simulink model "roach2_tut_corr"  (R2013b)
settings: Solver=VariableStepDiscrete  SolverMode=SingleTasking  StartTime=0.0  StopTime=100  RelTol=1e-3
undefined symbols (not defined in the file): add_latency, addr_width, Bit, bitfield, BitWidth, bram_latency, burst_size, casper_library_scopes, conv_latency, data_width, DelayLen, fan_latency, FFTSize, FFTStage, getfield, increment, led, Location, Lower, mult_latency, mux_latency, n_bits, n_bits_data, n_inputs, n_streams, n_taps, neg_latency, negate_latency, nsamples, pfb_size, pulse_len, reset_period, ROACH, ROACH2, snapshot, sx475t, sync_period, sync_period_bits, Upper, UseCounter, Width
libraries: xbsIndex_r4 x24444, casper_library_misc x73, xbsReplacements_r4 x34, casper_library_delays x14, xps_library x7
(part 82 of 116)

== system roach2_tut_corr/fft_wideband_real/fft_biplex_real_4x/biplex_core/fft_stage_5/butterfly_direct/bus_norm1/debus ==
  bus_in : Inport
  reinterpret{1..16} (16 alike) : xbsIndex_r4/Reinterpret  force_arith_type=on  arith_type="Signed  (2's comp)"  force_bin_pt=on  bin_pt=18  block_type=reinterpret
  slice1 : xbsIndex_r4/Slice  nbits=20  boolean_output=off  mode=Upper Bit Location + Width  bit1=-300  base1=MSB of Input  bit0=0  base0=LSB of Input  dbl_ovrd=off  block_type=slice
  slice10 : xbsIndex_r4/Slice  nbits=20  boolean_output=off  mode=Upper Bit Location + Width  bit1=-120  base1=MSB of Input  bit0=0  base0=LSB of Input  dbl_ovrd=off  block_type=slice
  slice11 : xbsIndex_r4/Slice  nbits=20  boolean_output=off  mode=Upper Bit Location + Width  bit1=-100  base1=MSB of Input  bit0=0  base0=LSB of Input  dbl_ovrd=off  block_type=slice
  slice12 : xbsIndex_r4/Slice  nbits=20  boolean_output=off  mode=Upper Bit Location + Width  bit1=-80  base1=MSB of Input  bit0=0  base0=LSB of Input  dbl_ovrd=off  block_type=slice
  slice13 : xbsIndex_r4/Slice  nbits=20  boolean_output=off  mode=Upper Bit Location + Width  bit1=-60  base1=MSB of Input  bit0=0  base0=LSB of Input  dbl_ovrd=off  block_type=slice
  slice14 : xbsIndex_r4/Slice  nbits=20  boolean_output=off  mode=Upper Bit Location + Width  bit1=-40  base1=MSB of Input  bit0=0  base0=LSB of Input  dbl_ovrd=off  block_type=slice
  slice15 : xbsIndex_r4/Slice  nbits=20  boolean_output=off  mode=Upper Bit Location + Width  bit1=-20  base1=MSB of Input  bit0=0  base0=LSB of Input  dbl_ovrd=off  block_type=slice
  slice16 : xbsIndex_r4/Slice  nbits=20  boolean_output=off  mode=Upper Bit Location + Width  bit1=0  base1=MSB of Input  bit0=0  base0=LSB of Input  dbl_ovrd=off  block_type=slice
  slice2 : xbsIndex_r4/Slice  nbits=20  boolean_output=off  mode=Upper Bit Location + Width  bit1=-280  base1=MSB of Input  bit0=0  base0=LSB of Input  dbl_ovrd=off  block_type=slice
  slice3 : xbsIndex_r4/Slice  nbits=20  boolean_output=off  mode=Upper Bit Location + Width  bit1=-260  base1=MSB of Input  bit0=0  base0=LSB of Input  dbl_ovrd=off  block_type=slice
  slice4 : xbsIndex_r4/Slice  nbits=20  boolean_output=off  mode=Upper Bit Location + Width  bit1=-240  base1=MSB of Input  bit0=0  base0=LSB of Input  dbl_ovrd=off  block_type=slice
  slice5 : xbsIndex_r4/Slice  nbits=20  boolean_output=off  mode=Upper Bit Location + Width  bit1=-220  base1=MSB of Input  bit0=0  base0=LSB of Input  dbl_ovrd=off  block_type=slice
  slice6 : xbsIndex_r4/Slice  nbits=20  boolean_output=off  mode=Upper Bit Location + Width  bit1=-200  base1=MSB of Input  bit0=0  base0=LSB of Input  dbl_ovrd=off  block_type=slice
  slice7 : xbsIndex_r4/Slice  nbits=20  boolean_output=off  mode=Upper Bit Location + Width  bit1=-180  base1=MSB of Input  bit0=0  base0=LSB of Input  dbl_ovrd=off  block_type=slice
  slice8 : xbsIndex_r4/Slice  nbits=20  boolean_output=off  mode=Upper Bit Location + Width  bit1=-160  base1=MSB of Input  bit0=0  base0=LSB of Input  dbl_ovrd=off  block_type=slice
  slice9 : xbsIndex_r4/Slice  nbits=20  boolean_output=off  mode=Upper Bit Location + Width  bit1=-140  base1=MSB of Input  bit0=0  base0=LSB of Input  dbl_ovrd=off  block_type=slice
  msb_out16 : Outport
  out15 : Outport  Port=2
  out14 : Outport  Port=3
  out13 : Outport  Port=4
  out12 : Outport  Port=5
  out11 : Outport  Port=6
  out10 : Outport  Port=7
  out9 : Outport  Port=8
  out8 : Outport  Port=9
  out7 : Outport  Port=10
  out6 : Outport  Port=11
  out5 : Outport  Port=12
  out4 : Outport  Port=13
  out3 : Outport  Port=14
  out2 : Outport  Port=15
  lsb_out1 : Outport  Port=16
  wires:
  bus_in/1 -> slice16/1, slice15/1, slice14/1, slice13/1, slice12/1, slice11/1, slice10/1, slice9/1, slice8/1, slice7/1, slice6/1, slice5/1, slice4/1, slice3/1, slice2/1, slice1/1
  slice16/1 -> reinterpret16/1
  reinterpret16/1 -> msb_out16/1
  slice15/1 -> reinterpret15/1
  reinterpret15/1 -> out15/1
  slice14/1 -> reinterpret14/1
  reinterpret14/1 -> out14/1
  slice13/1 -> reinterpret13/1
  reinterpret13/1 -> out13/1
  slice12/1 -> reinterpret12/1
  reinterpret12/1 -> out12/1
  slice11/1 -> reinterpret11/1
  reinterpret11/1 -> out11/1
  slice10/1 -> reinterpret10/1
  reinterpret10/1 -> out10/1
  slice9/1 -> reinterpret9/1
  reinterpret9/1 -> out9/1
  slice8/1 -> reinterpret8/1
  reinterpret8/1 -> out8/1
  slice7/1 -> reinterpret7/1
  reinterpret7/1 -> out7/1
  slice6/1 -> reinterpret6/1
  reinterpret6/1 -> out6/1
  slice5/1 -> reinterpret5/1
  reinterpret5/1 -> out5/1
  slice4/1 -> reinterpret4/1
  reinterpret4/1 -> out4/1
  slice3/1 -> reinterpret3/1
  reinterpret3/1 -> out3/1
  slice2/1 -> reinterpret2/1
  reinterpret2/1 -> out2/1
  slice1/1 -> reinterpret1/1
  reinterpret1/1 -> lsb_out1/1

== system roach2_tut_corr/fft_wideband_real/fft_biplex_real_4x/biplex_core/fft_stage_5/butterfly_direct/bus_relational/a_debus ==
  bus_in : Inport
  reinterpret1 : xbsIndex_r4/Reinterpret  force_arith_type=on  arith_type=Unsigned  force_bin_pt=on  bin_pt=0  block_type=reinterpret
  slice1 : xbsIndex_r4/Slice  nbits=4  boolean_output=off  mode=Upper Bit Location + Width  bit1=0  base1=MSB of Input  bit0=0  base0=LSB of Input  dbl_ovrd=off  block_type=slice
  msb_lsb_out1 : Outport
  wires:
  bus_in/1 -> slice1/1
  slice1/1 -> reinterpret1/1
  reinterpret1/1 -> msb_lsb_out1/1

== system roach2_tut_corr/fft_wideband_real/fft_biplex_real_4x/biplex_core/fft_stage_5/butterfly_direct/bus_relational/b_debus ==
  bus_in : Inport
  reinterpret{1..4} (4 alike) : xbsIndex_r4/Reinterpret  force_arith_type=on  arith_type=Unsigned  force_bin_pt=on  bin_pt=0  block_type=reinterpret
  slice1 : xbsIndex_r4/Slice  nbits=4  boolean_output=off  mode=Upper Bit Location + Width  bit1=-12  base1=MSB of Input  bit0=0  base0=LSB of Input  dbl_ovrd=off  block_type=slice
  slice2 : xbsIndex_r4/Slice  nbits=4  boolean_output=off  mode=Upper Bit Location + Width  bit1=-8  base1=MSB of Input  bit0=0  base0=LSB of Input  dbl_ovrd=off  block_type=slice
  slice3 : xbsIndex_r4/Slice  nbits=4  boolean_output=off  mode=Upper Bit Location + Width  bit1=-4  base1=MSB of Input  bit0=0  base0=LSB of Input  dbl_ovrd=off  block_type=slice
  slice4 : xbsIndex_r4/Slice  nbits=4  boolean_output=off  mode=Upper Bit Location + Width  bit1=0  base1=MSB of Input  bit0=0  base0=LSB of Input  dbl_ovrd=off  block_type=slice
  msb_out4 : Outport
  out3 : Outport  Port=2
  out2 : Outport  Port=3
  lsb_out1 : Outport  Port=4
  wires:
  bus_in/1 -> slice4/1, slice3/1, slice2/1, slice1/1
  slice4/1 -> reinterpret4/1
  reinterpret4/1 -> msb_out4/1
  slice3/1 -> reinterpret3/1
  reinterpret3/1 -> out3/1
  slice2/1 -> reinterpret2/1
  reinterpret2/1 -> out2/1
  slice1/1 -> reinterpret1/1
  reinterpret1/1 -> lsb_out1/1

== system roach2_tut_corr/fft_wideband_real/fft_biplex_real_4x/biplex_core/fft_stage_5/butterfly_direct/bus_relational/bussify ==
  in1 : Inport
  in2 : Inport  Port=2
  in3 : Inport  Port=3
  in4 : Inport  Port=4
  concatenate : xbsIndex_r4/Concat  num_inputs=4  dbl_ovrd=off  block_type=concat
  reinterpret{1..4} (4 alike) : xbsIndex_r4/Reinterpret  force_arith_type=on  arith_type=Unsigned  force_bin_pt=on  bin_pt=0  block_type=reinterpret
  bus_out : Outport
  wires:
  concatenate/1 -> bus_out/1
  in1/1 -> reinterpret1/1
  reinterpret1/1 -> concatenate/1
  in2/1 -> reinterpret2/1
  reinterpret2/1 -> concatenate/2
  in3/1 -> reinterpret3/1
  reinterpret3/1 -> concatenate/3
  in4/1 -> reinterpret4/1
  reinterpret4/1 -> concatenate/4

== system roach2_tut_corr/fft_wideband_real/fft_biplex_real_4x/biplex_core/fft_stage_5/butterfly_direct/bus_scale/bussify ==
  in1 : Inport
  in2 : Inport  Port=2
  in3 : Inport  Port=3
  in4 : Inport  Port=4
  in5 : Inport  Port=5
  in6 : Inport  Port=6
  in7 : Inport  Port=7
  in8 : Inport  Port=8
  in9 : Inport  Port=9
  in10 : Inport  Port=10
  in11 : Inport  Port=11
  in12 : Inport  Port=12
  in13 : Inport  Port=13
  in14 : Inport  Port=14
  in15 : Inport  Port=15
  in16 : Inport  Port=16
  concatenate : xbsIndex_r4/Concat  num_inputs=16  dbl_ovrd=off  block_type=concat
  reinterpret{1..16} (16 alike) : xbsIndex_r4/Reinterpret  force_arith_type=on  arith_type=Unsigned  force_bin_pt=on  bin_pt=0  block_type=reinterpret
  bus_out : Outport
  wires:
  concatenate/1 -> bus_out/1
  in1/1 -> reinterpret1/1
  reinterpret1/1 -> concatenate/1
  in2/1 -> reinterpret2/1
  reinterpret2/1 -> concatenate/2
  in3/1 -> reinterpret3/1
  reinterpret3/1 -> concatenate/3
  in4/1 -> reinterpret4/1
  reinterpret4/1 -> concatenate/4
  in5/1 -> reinterpret5/1
  reinterpret5/1 -> concatenate/5
  in6/1 -> reinterpret6/1
  reinterpret6/1 -> concatenate/6
  in7/1 -> reinterpret7/1
  reinterpret7/1 -> concatenate/7
  in8/1 -> reinterpret8/1
  reinterpret8/1 -> concatenate/8
  in9/1 -> reinterpret9/1
  reinterpret9/1 -> concatenate/9
  in10/1 -> reinterpret10/1
  reinterpret10/1 -> concatenate/10
  in11/1 -> reinterpret11/1
  reinterpret11/1 -> concatenate/11
  in12/1 -> reinterpret12/1
  reinterpret12/1 -> concatenate/12
  in13/1 -> reinterpret13/1
  reinterpret13/1 -> concatenate/13
  in14/1 -> reinterpret14/1
  reinterpret14/1 -> concatenate/14
  in15/1 -> reinterpret15/1
  reinterpret15/1 -> concatenate/15
  in16/1 -> reinterpret16/1
  reinterpret16/1 -> concatenate/16

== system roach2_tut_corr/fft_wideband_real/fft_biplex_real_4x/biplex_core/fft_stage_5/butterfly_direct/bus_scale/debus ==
  bus_in : Inport
  reinterpret{1..16} (16 alike) : xbsIndex_r4/Reinterpret  force_arith_type=on  arith_type="Signed  (2's comp)"  force_bin_pt=on  bin_pt=17  block_type=reinterpret
  slice1 : xbsIndex_r4/Slice  nbits=20  boolean_output=off  mode=Upper Bit Location + Width  bit1=-300  base1=MSB of Input  bit0=0  base0=LSB of Input  dbl_ovrd=off  block_type=slice
  slice10 : xbsIndex_r4/Slice  nbits=20  boolean_output=off  mode=Upper Bit Location + Width  bit1=-120  base1=MSB of Input  bit0=0  base0=LSB of Input  dbl_ovrd=off  block_type=slice
  slice11 : xbsIndex_r4/Slice  nbits=20  boolean_output=off  mode=Upper Bit Location + Width  bit1=-100  base1=MSB of Input  bit0=0  base0=LSB of Input  dbl_ovrd=off  block_type=slice
  slice12 : xbsIndex_r4/Slice  nbits=20  boolean_output=off  mode=Upper Bit Location + Width  bit1=-80  base1=MSB of Input  bit0=0  base0=LSB of Input  dbl_ovrd=off  block_type=slice
  slice13 : xbsIndex_r4/Slice  nbits=20  boolean_output=off  mode=Upper Bit Location + Width  bit1=-60  base1=MSB of Input  bit0=0  base0=LSB of Input  dbl_ovrd=off  block_type=slice
  slice14 : xbsIndex_r4/Slice  nbits=20  boolean_output=off  mode=Upper Bit Location + Width  bit1=-40  base1=MSB of Input  bit0=0  base0=LSB of Input  dbl_ovrd=off  block_type=slice
  slice15 : xbsIndex_r4/Slice  nbits=20  boolean_output=off  mode=Upper Bit Location + Width  bit1=-20  base1=MSB of Input  bit0=0  base0=LSB of Input  dbl_ovrd=off  block_type=slice
  slice16 : xbsIndex_r4/Slice  nbits=20  boolean_output=off  mode=Upper Bit Location + Width  bit1=0  base1=MSB of Input  bit0=0  base0=LSB of Input  dbl_ovrd=off  block_type=slice
  slice2 : xbsIndex_r4/Slice  nbits=20  boolean_output=off  mode=Upper Bit Location + Width  bit1=-280  base1=MSB of Input  bit0=0  base0=LSB of Input  dbl_ovrd=off  block_type=slice
  slice3 : xbsIndex_r4/Slice  nbits=20  boolean_output=off  mode=Upper Bit Location + Width  bit1=-260  base1=MSB of Input  bit0=0  base0=LSB of Input  dbl_ovrd=off  block_type=slice
  slice4 : xbsIndex_r4/Slice  nbits=20  boolean_output=off  mode=Upper Bit Location + Width  bit1=-240  base1=MSB of Input  bit0=0  base0=LSB of Input  dbl_ovrd=off  block_type=slice
  slice5 : xbsIndex_r4/Slice  nbits=20  boolean_output=off  mode=Upper Bit Location + Width  bit1=-220  base1=MSB of Input  bit0=0  base0=LSB of Input  dbl_ovrd=off  block_type=slice
  slice6 : xbsIndex_r4/Slice  nbits=20  boolean_output=off  mode=Upper Bit Location + Width  bit1=-200  base1=MSB of Input  bit0=0  base0=LSB of Input  dbl_ovrd=off  block_type=slice
  slice7 : xbsIndex_r4/Slice  nbits=20  boolean_output=off  mode=Upper Bit Location + Width  bit1=-180  base1=MSB of Input  bit0=0  base0=LSB of Input  dbl_ovrd=off  block_type=slice
  slice8 : xbsIndex_r4/Slice  nbits=20  boolean_output=off  mode=Upper Bit Location + Width  bit1=-160  base1=MSB of Input  bit0=0  base0=LSB of Input  dbl_ovrd=off  block_type=slice
  slice9 : xbsIndex_r4/Slice  nbits=20  boolean_output=off  mode=Upper Bit Location + Width  bit1=-140  base1=MSB of Input  bit0=0  base0=LSB of Input  dbl_ovrd=off  block_type=slice
  msb_out16 : Outport
  out15 : Outport  Port=2
  out14 : Outport  Port=3
  out13 : Outport  Port=4
  out12 : Outport  Port=5
  out11 : Outport  Port=6
  out10 : Outport  Port=7
  out9 : Outport  Port=8
  out8 : Outport  Port=9
  out7 : Outport  Port=10
  out6 : Outport  Port=11
  out5 : Outport  Port=12
  out4 : Outport  Port=13
  out3 : Outport  Port=14
  out2 : Outport  Port=15
  lsb_out1 : Outport  Port=16
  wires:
  bus_in/1 -> slice16/1, slice15/1, slice14/1, slice13/1, slice12/1, slice11/1, slice10/1, slice9/1, slice8/1, slice7/1, slice6/1, slice5/1, slice4/1, slice3/1, slice2/1, slice1/1
  slice16/1 -> reinterpret16/1
  reinterpret16/1 -> msb_out16/1
  slice15/1 -> reinterpret15/1
  reinterpret15/1 -> out15/1
  slice14/1 -> reinterpret14/1
  reinterpret14/1 -> out14/1
  slice13/1 -> reinterpret13/1
  reinterpret13/1 -> out13/1
  slice12/1 -> reinterpret12/1
  reinterpret12/1 -> out12/1
  slice11/1 -> reinterpret11/1
  reinterpret11/1 -> out11/1
  slice10/1 -> reinterpret10/1
  reinterpret10/1 -> out10/1
  slice9/1 -> reinterpret9/1
  reinterpret9/1 -> out9/1
  slice8/1 -> reinterpret8/1
  reinterpret8/1 -> out8/1
  slice7/1 -> reinterpret7/1
  reinterpret7/1 -> out7/1
  slice6/1 -> reinterpret6/1
  reinterpret6/1 -> out6/1
  slice5/1 -> reinterpret5/1
  reinterpret5/1 -> out5/1
  slice4/1 -> reinterpret4/1
  reinterpret4/1 -> out4/1
  slice3/1 -> reinterpret3/1
  reinterpret3/1 -> out3/1
  slice2/1 -> reinterpret2/1
  reinterpret2/1 -> out2/1
  slice1/1 -> reinterpret1/1
  reinterpret1/1 -> lsb_out1/1

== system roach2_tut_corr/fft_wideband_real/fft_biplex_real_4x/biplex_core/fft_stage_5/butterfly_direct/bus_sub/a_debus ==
  bus_in : Inport
  reinterpret{1..8} (8 alike) : xbsIndex_r4/Reinterpret  force_arith_type=on  arith_type="Signed  (2's comp)"  force_bin_pt=on  bin_pt=17  block_type=reinterpret
  slice1 : xbsIndex_r4/Slice  nbits=18  boolean_output=off  mode=Upper Bit Location + Width  bit1=-126  base1=MSB of Input  bit0=0  base0=LSB of Input  dbl_ovrd=off  block_type=slice
  slice2 : xbsIndex_r4/Slice  nbits=18  boolean_output=off  mode=Upper Bit Location + Width  bit1=-108  base1=MSB of Input  bit0=0  base0=LSB of Input  dbl_ovrd=off  block_type=slice
  slice3 : xbsIndex_r4/Slice  nbits=18  boolean_output=off  mode=Upper Bit Location + Width  bit1=-90  base1=MSB of Input  bit0=0  base0=LSB of Input  dbl_ovrd=off  block_type=slice
  slice4 : xbsIndex_r4/Slice  nbits=18  boolean_output=off  mode=Upper Bit Location + Width  bit1=-72  base1=MSB of Input  bit0=0  base0=LSB of Input  dbl_ovrd=off  block_type=slice
  slice5 : xbsIndex_r4/Slice  nbits=18  boolean_output=off  mode=Upper Bit Location + Width  bit1=-54  base1=MSB of Input  bit0=0  base0=LSB of Input  dbl_ovrd=off  block_type=slice
  slice6 : xbsIndex_r4/Slice  nbits=18  boolean_output=off  mode=Upper Bit Location + Width  bit1=-36  base1=MSB of Input  bit0=0  base0=LSB of Input  dbl_ovrd=off  block_type=slice
  slice7 : xbsIndex_r4/Slice  nbits=18  boolean_output=off  mode=Upper Bit Location + Width  bit1=-18  base1=MSB of Input  bit0=0  base0=LSB of Input  dbl_ovrd=off  block_type=slice
  slice8 : xbsIndex_r4/Slice  nbits=18  boolean_output=off  mode=Upper Bit Location + Width  bit1=0  base1=MSB of Input  bit0=0  base0=LSB of Input  dbl_ovrd=off  block_type=slice
  msb_out8 : Outport
  out7 : Outport  Port=2
  out6 : Outport  Port=3
  out5 : Outport  Port=4
  out4 : Outport  Port=5
  out3 : Outport  Port=6
  out2 : Outport  Port=7
  lsb_out1 : Outport  Port=8
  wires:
  bus_in/1 -> slice8/1, slice7/1, slice6/1, slice5/1, slice4/1, slice3/1, slice2/1, slice1/1
  slice8/1 -> reinterpret8/1
  reinterpret8/1 -> msb_out8/1
  slice7/1 -> reinterpret7/1
  reinterpret7/1 -> out7/1
  slice6/1 -> reinterpret6/1
  reinterpret6/1 -> out6/1
  slice5/1 -> reinterpret5/1
  reinterpret5/1 -> out5/1
  slice4/1 -> reinterpret4/1
  reinterpret4/1 -> out4/1
  slice3/1 -> reinterpret3/1
  reinterpret3/1 -> out3/1
  slice2/1 -> reinterpret2/1
  reinterpret2/1 -> out2/1
  slice1/1 -> reinterpret1/1
  reinterpret1/1 -> lsb_out1/1

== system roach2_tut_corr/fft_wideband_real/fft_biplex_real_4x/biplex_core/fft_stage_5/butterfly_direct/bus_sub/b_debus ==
  bus_in : Inport
  reinterpret{1..8} (8 alike) : xbsIndex_r4/Reinterpret  force_arith_type=on  arith_type="Signed  (2's comp)"  force_bin_pt=on  bin_pt=17  block_type=reinterpret
  slice1 : xbsIndex_r4/Slice  nbits=19  boolean_output=off  mode=Upper Bit Location + Width  bit1=-133  base1=MSB of Input  bit0=0  base0=LSB of Input  dbl_ovrd=off  block_type=slice
  slice2 : xbsIndex_r4/Slice  nbits=19  boolean_output=off  mode=Upper Bit Location + Width  bit1=-114  base1=MSB of Input  bit0=0  base0=LSB of Input  dbl_ovrd=off  block_type=slice
  slice3 : xbsIndex_r4/Slice  nbits=19  boolean_output=off  mode=Upper Bit Location + Width  bit1=-95  base1=MSB of Input  bit0=0  base0=LSB of Input  dbl_ovrd=off  block_type=slice
  slice4 : xbsIndex_r4/Slice  nbits=19  boolean_output=off  mode=Upper Bit Location + Width  bit1=-76  base1=MSB of Input  bit0=0  base0=LSB of Input  dbl_ovrd=off  block_type=slice
  slice5 : xbsIndex_r4/Slice  nbits=19  boolean_output=off  mode=Upper Bit Location + Width  bit1=-57  base1=MSB of Input  bit0=0  base0=LSB of Input  dbl_ovrd=off  block_type=slice
  slice6 : xbsIndex_r4/Slice  nbits=19  boolean_output=off  mode=Upper Bit Location + Width  bit1=-38  base1=MSB of Input  bit0=0  base0=LSB of Input  dbl_ovrd=off  block_type=slice
  slice7 : xbsIndex_r4/Slice  nbits=19  boolean_output=off  mode=Upper Bit Location + Width  bit1=-19  base1=MSB of Input  bit0=0  base0=LSB of Input  dbl_ovrd=off  block_type=slice
  slice8 : xbsIndex_r4/Slice  nbits=19  boolean_output=off  mode=Upper Bit Location + Width  bit1=0  base1=MSB of Input  bit0=0  base0=LSB of Input  dbl_ovrd=off  block_type=slice
  msb_out8 : Outport
  out7 : Outport  Port=2
  out6 : Outport  Port=3
  out5 : Outport  Port=4
  out4 : Outport  Port=5
  out3 : Outport  Port=6
  out2 : Outport  Port=7
  lsb_out1 : Outport  Port=8
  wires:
  bus_in/1 -> slice8/1, slice7/1, slice6/1, slice5/1, slice4/1, slice3/1, slice2/1, slice1/1
  slice8/1 -> reinterpret8/1
  reinterpret8/1 -> msb_out8/1
  slice7/1 -> reinterpret7/1
  reinterpret7/1 -> out7/1
  slice6/1 -> reinterpret6/1
  reinterpret6/1 -> out6/1
  slice5/1 -> reinterpret5/1
  reinterpret5/1 -> out5/1
  slice4/1 -> reinterpret4/1
  reinterpret4/1 -> out4/1
  slice3/1 -> reinterpret3/1
  reinterpret3/1 -> out3/1
  slice2/1 -> reinterpret2/1
  reinterpret2/1 -> out2/1
  slice1/1 -> reinterpret1/1
  reinterpret1/1 -> lsb_out1/1

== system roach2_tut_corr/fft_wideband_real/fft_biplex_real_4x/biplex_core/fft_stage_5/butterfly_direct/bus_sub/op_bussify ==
  in1 : Inport
  in2 : Inport  Port=2
  in3 : Inport  Port=3
  in4 : Inport  Port=4
  in5 : Inport  Port=5
  in6 : Inport  Port=6
  in7 : Inport  Port=7
  in8 : Inport  Port=8
  concatenate : xbsIndex_r4/Concat  num_inputs=8  dbl_ovrd=off  block_type=concat
  reinterpret{1..8} (8 alike) : xbsIndex_r4/Reinterpret  force_arith_type=on  arith_type=Unsigned  force_bin_pt=on  bin_pt=0  block_type=reinterpret
  bus_out : Outport
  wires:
  concatenate/1 -> bus_out/1
  in1/1 -> reinterpret1/1
  reinterpret1/1 -> concatenate/1
  in2/1 -> reinterpret2/1
  reinterpret2/1 -> concatenate/2
  in3/1 -> reinterpret3/1
  reinterpret3/1 -> concatenate/3
  in4/1 -> reinterpret4/1
  reinterpret4/1 -> concatenate/4
  in5/1 -> reinterpret5/1
  reinterpret5/1 -> concatenate/5
  in6/1 -> reinterpret6/1
  reinterpret6/1 -> concatenate/6
  in7/1 -> reinterpret7/1
  reinterpret7/1 -> concatenate/7
  in8/1 -> reinterpret8/1
  reinterpret8/1 -> concatenate/8

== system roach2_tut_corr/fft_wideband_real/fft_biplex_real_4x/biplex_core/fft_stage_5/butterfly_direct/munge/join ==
  in1 : Inport
  in2 : Inport  Port=2
  in3 : Inport  Port=3
  in4 : Inport  Port=4
  in5 : Inport  Port=5
  in6 : Inport  Port=6
  in7 : Inport  Port=7
  in8 : Inport  Port=8
  concatenate : xbsIndex_r4/Concat  num_inputs=8  dbl_ovrd=off  block_type=concat
  reinterpret{1..8} (8 alike) : xbsIndex_r4/Reinterpret  force_arith_type=on  arith_type=Unsigned  force_bin_pt=on  bin_pt=0  block_type=reinterpret
  bus_out : Outport
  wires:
  concatenate/1 -> bus_out/1
  in1/1 -> reinterpret1/1
  reinterpret1/1 -> concatenate/1
  in2/1 -> reinterpret2/1
  reinterpret2/1 -> concatenate/2
  in3/1 -> reinterpret3/1
  reinterpret3/1 -> concatenate/3
  in4/1 -> reinterpret4/1
  reinterpret4/1 -> concatenate/4
  in5/1 -> reinterpret5/1
  reinterpret5/1 -> concatenate/5
  in6/1 -> reinterpret6/1
  reinterpret6/1 -> concatenate/6
  in7/1 -> reinterpret7/1
  reinterpret7/1 -> concatenate/7
  in8/1 -> reinterpret8/1
  reinterpret8/1 -> concatenate/8

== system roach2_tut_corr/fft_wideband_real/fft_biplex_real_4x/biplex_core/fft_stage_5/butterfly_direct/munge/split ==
  bus_in : Inport
  reinterpret{1..8} (8 alike) : xbsIndex_r4/Reinterpret  force_arith_type=on  arith_type=Unsigned  force_bin_pt=on  bin_pt=0  block_type=reinterpret
  slice1 : xbsIndex_r4/Slice  nbits=2  boolean_output=off  mode=Upper Bit Location + Width  bit1=-14  base1=MSB of Input  bit0=0  base0=LSB of Input  dbl_ovrd=off  block_type=slice
  slice2 : xbsIndex_r4/Slice  nbits=2  boolean_output=off  mode=Upper Bit Location + Width  bit1=-12  base1=MSB of Input  bit0=0  base0=LSB of Input  dbl_ovrd=off  block_type=slice
  slice3 : xbsIndex_r4/Slice  nbits=2  boolean_output=off  mode=Upper Bit Location + Width  bit1=-10  base1=MSB of Input  bit0=0  base0=LSB of Input  dbl_ovrd=off  block_type=slice
  slice4 : xbsIndex_r4/Slice  nbits=2  boolean_output=off  mode=Upper Bit Location + Width  bit1=-8  base1=MSB of Input  bit0=0  base0=LSB of Input  dbl_ovrd=off  block_type=slice
  slice5 : xbsIndex_r4/Slice  nbits=2  boolean_output=off  mode=Upper Bit Location + Width  bit1=-6  base1=MSB of Input  bit0=0  base0=LSB of Input  dbl_ovrd=off  block_type=slice
  slice6 : xbsIndex_r4/Slice  nbits=2  boolean_output=off  mode=Upper Bit Location + Width  bit1=-4  base1=MSB of Input  bit0=0  base0=LSB of Input  dbl_ovrd=off  block_type=slice
  slice7 : xbsIndex_r4/Slice  nbits=2  boolean_output=off  mode=Upper Bit Location + Width  bit1=-2  base1=MSB of Input  bit0=0  base0=LSB of Input  dbl_ovrd=off  block_type=slice
  slice8 : xbsIndex_r4/Slice  nbits=2  boolean_output=off  mode=Upper Bit Location + Width  bit1=0  base1=MSB of Input  bit0=0  base0=LSB of Input  dbl_ovrd=off  block_type=slice
  msb_out8 : Outport
  out7 : Outport  Port=2
  out6 : Outport  Port=3
  out5 : Outport  Port=4
  out4 : Outport  Port=5
  out3 : Outport  Port=6
  out2 : Outport  Port=7
  lsb_out1 : Outport  Port=8
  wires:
  bus_in/1 -> slice8/1, slice7/1, slice6/1, slice5/1, slice4/1, slice3/1, slice2/1, slice1/1
  slice8/1 -> reinterpret8/1
  reinterpret8/1 -> msb_out8/1
  slice7/1 -> reinterpret7/1
  reinterpret7/1 -> out7/1
  slice6/1 -> reinterpret6/1
  reinterpret6/1 -> out6/1
  slice5/1 -> reinterpret5/1
  reinterpret5/1 -> out5/1
  slice4/1 -> reinterpret4/1
  reinterpret4/1 -> out4/1
  slice3/1 -> reinterpret3/1
  reinterpret3/1 -> out3/1
  slice2/1 -> reinterpret2/1
  reinterpret2/1 -> out2/1
  slice1/1 -> reinterpret1/1
  reinterpret1/1 -> lsb_out1/1

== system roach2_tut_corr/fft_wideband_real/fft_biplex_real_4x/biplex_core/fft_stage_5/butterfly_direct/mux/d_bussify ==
  in1 : Inport
  in2 : Inport  Port=2
  in3 : Inport  Port=3
  in4 : Inport  Port=4
  in5 : Inport  Port=5
  in6 : Inport  Port=6
  in7 : Inport  Port=7
  in8 : Inport  Port=8
  in9 : Inport  Port=9
  in10 : Inport  Port=10
  in11 : Inport  Port=11
  in12 : Inport  Port=12
  in13 : Inport  Port=13
  in14 : Inport  Port=14
  in15 : Inport  Port=15
  in16 : Inport  Port=16
  concatenate : xbsIndex_r4/Concat  num_inputs=16  dbl_ovrd=off  block_type=concat
  reinterpret{1..16} (16 alike) : xbsIndex_r4/Reinterpret  force_arith_type=on  arith_type=Unsigned  force_bin_pt=on  bin_pt=0  block_type=reinterpret
  bus_out : Outport
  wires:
  concatenate/1 -> bus_out/1
  in1/1 -> reinterpret1/1
  reinterpret1/1 -> concatenate/1
  in2/1 -> reinterpret2/1
  reinterpret2/1 -> concatenate/2
  in3/1 -> reinterpret3/1
  reinterpret3/1 -> concatenate/3
  in4/1 -> reinterpret4/1
  reinterpret4/1 -> concatenate/4
  in5/1 -> reinterpret5/1
  reinterpret5/1 -> concatenate/5
  in6/1 -> reinterpret6/1
  reinterpret6/1 -> concatenate/6
  in7/1 -> reinterpret7/1
  reinterpret7/1 -> concatenate/7
  in8/1 -> reinterpret8/1
  reinterpret8/1 -> concatenate/8
  in9/1 -> reinterpret9/1
  reinterpret9/1 -> concatenate/9
  in10/1 -> reinterpret10/1
  reinterpret10/1 -> concatenate/10
  in11/1 -> reinterpret11/1
  reinterpret11/1 -> concatenate/11
  in12/1 -> reinterpret12/1
  reinterpret12/1 -> concatenate/12
  in13/1 -> reinterpret13/1
  reinterpret13/1 -> concatenate/13
  in14/1 -> reinterpret14/1
  reinterpret14/1 -> concatenate/14
  in15/1 -> reinterpret15/1
  reinterpret15/1 -> concatenate/15
  in16/1 -> reinterpret16/1
  reinterpret16/1 -> concatenate/16

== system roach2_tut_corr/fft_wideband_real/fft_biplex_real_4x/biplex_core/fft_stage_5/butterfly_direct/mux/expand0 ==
  bus_in : Inport
  reinterpret{1..16} (16 alike) : xbsIndex_r4/Reinterpret  force_arith_type=on  arith_type=Unsigned  force_bin_pt=on  bin_pt=0  block_type=reinterpret
  slice1 : xbsIndex_r4/Slice  nbits=21  boolean_output=off  mode=Upper Bit Location + Width  bit1=-315  base1=MSB of Input  bit0=0  base0=LSB of Input  dbl_ovrd=off  block_type=slice
  slice10 : xbsIndex_r4/Slice  nbits=21  boolean_output=off  mode=Upper Bit Location + Width  bit1=-126  base1=MSB of Input  bit0=0  base0=LSB of Input  dbl_ovrd=off  block_type=slice
  slice11 : xbsIndex_r4/Slice  nbits=21  boolean_output=off  mode=Upper Bit Location + Width  bit1=-105  base1=MSB of Input  bit0=0  base0=LSB of Input  dbl_ovrd=off  block_type=slice
  slice12 : xbsIndex_r4/Slice  nbits=21  boolean_output=off  mode=Upper Bit Location + Width  bit1=-84  base1=MSB of Input  bit0=0  base0=LSB of Input  dbl_ovrd=off  block_type=slice
  slice13 : xbsIndex_r4/Slice  nbits=21  boolean_output=off  mode=Upper Bit Location + Width  bit1=-63  base1=MSB of Input  bit0=0  base0=LSB of Input  dbl_ovrd=off  block_type=slice
  slice14 : xbsIndex_r4/Slice  nbits=21  boolean_output=off  mode=Upper Bit Location + Width  bit1=-42  base1=MSB of Input  bit0=0  base0=LSB of Input  dbl_ovrd=off  block_type=slice
  slice15 : xbsIndex_r4/Slice  nbits=21  boolean_output=off  mode=Upper Bit Location + Width  bit1=-21  base1=MSB of Input  bit0=0  base0=LSB of Input  dbl_ovrd=off  block_type=slice
  slice16 : xbsIndex_r4/Slice  nbits=21  boolean_output=off  mode=Upper Bit Location + Width  bit1=0  base1=MSB of Input  bit0=0  base0=LSB of Input  dbl_ovrd=off  block_type=slice
  slice2 : xbsIndex_r4/Slice  nbits=21  boolean_output=off  mode=Upper Bit Location + Width  bit1=-294  base1=MSB of Input  bit0=0  base0=LSB of Input  dbl_ovrd=off  block_type=slice
  slice3 : xbsIndex_r4/Slice  nbits=21  boolean_output=off  mode=Upper Bit Location + Width  bit1=-273  base1=MSB of Input  bit0=0  base0=LSB of Input  dbl_ovrd=off  block_type=slice
  slice4 : xbsIndex_r4/Slice  nbits=21  boolean_output=off  mode=Upper Bit Location + Width  bit1=-252  base1=MSB of Input  bit0=0  base0=LSB of Input  dbl_ovrd=off  block_type=slice
  slice5 : xbsIndex_r4/Slice  nbits=21  boolean_output=off  mode=Upper Bit Location + Width  bit1=-231  base1=MSB of Input  bit0=0  base0=LSB of Input  dbl_ovrd=off  block_type=slice
  slice6 : xbsIndex_r4/Slice  nbits=21  boolean_output=off  mode=Upper Bit Location + Width  bit1=-210  base1=MSB of Input  bit0=0  base0=LSB of Input  dbl_ovrd=off  block_type=slice
  slice7 : xbsIndex_r4/Slice  nbits=21  boolean_output=off  mode=Upper Bit Location + Width  bit1=-189  base1=MSB of Input  bit0=0  base0=LSB of Input  dbl_ovrd=off  block_type=slice
  slice8 : xbsIndex_r4/Slice  nbits=21  boolean_output=off  mode=Upper Bit Location + Width  bit1=-168  base1=MSB of Input  bit0=0  base0=LSB of Input  dbl_ovrd=off  block_type=slice
  slice9 : xbsIndex_r4/Slice  nbits=21  boolean_output=off  mode=Upper Bit Location + Width  bit1=-147  base1=MSB of Input  bit0=0  base0=LSB of Input  dbl_ovrd=off  block_type=slice
  msb_out16 : Outport
  out15 : Outport  Port=2
  out14 : Outport  Port=3
  out13 : Outport  Port=4
  out12 : Outport  Port=5
  out11 : Outport  Port=6
  out10 : Outport  Port=7
  out9 : Outport  Port=8
  out8 : Outport  Port=9
  out7 : Outport  Port=10
  out6 : Outport  Port=11
  out5 : Outport  Port=12
  out4 : Outport  Port=13
  out3 : Outport  Port=14
  out2 : Outport  Port=15
  lsb_out1 : Outport  Port=16
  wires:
  bus_in/1 -> slice16/1, slice15/1, slice14/1, slice13/1, slice12/1, slice11/1, slice10/1, slice9/1, slice8/1, slice7/1, slice6/1, slice5/1, slice4/1, slice3/1, slice2/1, slice1/1
  slice16/1 -> reinterpret16/1
  reinterpret16/1 -> msb_out16/1
  slice15/1 -> reinterpret15/1
  reinterpret15/1 -> out15/1
  slice14/1 -> reinterpret14/1
  reinterpret14/1 -> out14/1
  slice13/1 -> reinterpret13/1
  reinterpret13/1 -> out13/1
  slice12/1 -> reinterpret12/1
  reinterpret12/1 -> out12/1
  slice11/1 -> reinterpret11/1
  reinterpret11/1 -> out11/1
  slice10/1 -> reinterpret10/1
  reinterpret10/1 -> out10/1
  slice9/1 -> reinterpret9/1
  reinterpret9/1 -> out9/1
  slice8/1 -> reinterpret8/1
  reinterpret8/1 -> out8/1
  slice7/1 -> reinterpret7/1
  reinterpret7/1 -> out7/1
  slice6/1 -> reinterpret6/1
  reinterpret6/1 -> out6/1
  slice5/1 -> reinterpret5/1
  reinterpret5/1 -> out5/1
  slice4/1 -> reinterpret4/1
  reinterpret4/1 -> out4/1
  slice3/1 -> reinterpret3/1
  reinterpret3/1 -> out3/1
  slice2/1 -> reinterpret2/1
  reinterpret2/1 -> out2/1
  slice1/1 -> reinterpret1/1
  reinterpret1/1 -> lsb_out1/1

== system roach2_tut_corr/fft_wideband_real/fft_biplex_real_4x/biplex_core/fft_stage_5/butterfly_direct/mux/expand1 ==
  bus_in : Inport
  reinterpret{1..16} (16 alike) : xbsIndex_r4/Reinterpret  force_arith_type=on  arith_type=Unsigned  force_bin_pt=on  bin_pt=0  block_type=reinterpret
  slice1 : xbsIndex_r4/Slice  nbits=21  boolean_output=off  mode=Upper Bit Location + Width  bit1=-315  base1=MSB of Input  bit0=0  base0=LSB of Input  dbl_ovrd=off  block_type=slice
  slice10 : xbsIndex_r4/Slice  nbits=21  boolean_output=off  mode=Upper Bit Location + Width  bit1=-126  base1=MSB of Input  bit0=0  base0=LSB of Input  dbl_ovrd=off  block_type=slice
  slice11 : xbsIndex_r4/Slice  nbits=21  boolean_output=off  mode=Upper Bit Location + Width  bit1=-105  base1=MSB of Input  bit0=0  base0=LSB of Input  dbl_ovrd=off  block_type=slice
  slice12 : xbsIndex_r4/Slice  nbits=21  boolean_output=off  mode=Upper Bit Location + Width  bit1=-84  base1=MSB of Input  bit0=0  base0=LSB of Input  dbl_ovrd=off  block_type=slice
  slice13 : xbsIndex_r4/Slice  nbits=21  boolean_output=off  mode=Upper Bit Location + Width  bit1=-63  base1=MSB of Input  bit0=0  base0=LSB of Input  dbl_ovrd=off  block_type=slice
  slice14 : xbsIndex_r4/Slice  nbits=21  boolean_output=off  mode=Upper Bit Location + Width  bit1=-42  base1=MSB of Input  bit0=0  base0=LSB of Input  dbl_ovrd=off  block_type=slice
  slice15 : xbsIndex_r4/Slice  nbits=21  boolean_output=off  mode=Upper Bit Location + Width  bit1=-21  base1=MSB of Input  bit0=0  base0=LSB of Input  dbl_ovrd=off  block_type=slice
  slice16 : xbsIndex_r4/Slice  nbits=21  boolean_output=off  mode=Upper Bit Location + Width  bit1=0  base1=MSB of Input  bit0=0  base0=LSB of Input  dbl_ovrd=off  block_type=slice
  slice2 : xbsIndex_r4/Slice  nbits=21  boolean_output=off  mode=Upper Bit Location + Width  bit1=-294  base1=MSB of Input  bit0=0  base0=LSB of Input  dbl_ovrd=off  block_type=slice
  slice3 : xbsIndex_r4/Slice  nbits=21  boolean_output=off  mode=Upper Bit Location + Width  bit1=-273  base1=MSB of Input  bit0=0  base0=LSB of Input  dbl_ovrd=off  block_type=slice
  slice4 : xbsIndex_r4/Slice  nbits=21  boolean_output=off  mode=Upper Bit Location + Width  bit1=-252  base1=MSB of Input  bit0=0  base0=LSB of Input  dbl_ovrd=off  block_type=slice
  slice5 : xbsIndex_r4/Slice  nbits=21  boolean_output=off  mode=Upper Bit Location + Width  bit1=-231  base1=MSB of Input  bit0=0  base0=LSB of Input  dbl_ovrd=off  block_type=slice
  slice6 : xbsIndex_r4/Slice  nbits=21  boolean_output=off  mode=Upper Bit Location + Width  bit1=-210  base1=MSB of Input  bit0=0  base0=LSB of Input  dbl_ovrd=off  block_type=slice
  slice7 : xbsIndex_r4/Slice  nbits=21  boolean_output=off  mode=Upper Bit Location + Width  bit1=-189  base1=MSB of Input  bit0=0  base0=LSB of Input  dbl_ovrd=off  block_type=slice
  slice8 : xbsIndex_r4/Slice  nbits=21  boolean_output=off  mode=Upper Bit Location + Width  bit1=-168  base1=MSB of Input  bit0=0  base0=LSB of Input  dbl_ovrd=off  block_type=slice
  slice9 : xbsIndex_r4/Slice  nbits=21  boolean_output=off  mode=Upper Bit Location + Width  bit1=-147  base1=MSB of Input  bit0=0  base0=LSB of Input  dbl_ovrd=off  block_type=slice
  msb_out16 : Outport
  out15 : Outport  Port=2
  out14 : Outport  Port=3
  out13 : Outport  Port=4
  out12 : Outport  Port=5
  out11 : Outport  Port=6
  out10 : Outport  Port=7
  out9 : Outport  Port=8
  out8 : Outport  Port=9
  out7 : Outport  Port=10
  out6 : Outport  Port=11
  out5 : Outport  Port=12
  out4 : Outport  Port=13
  out3 : Outport  Port=14
  out2 : Outport  Port=15
  lsb_out1 : Outport  Port=16
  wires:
  bus_in/1 -> slice16/1, slice15/1, slice14/1, slice13/1, slice12/1, slice11/1, slice10/1, slice9/1, slice8/1, slice7/1, slice6/1, slice5/1, slice4/1, slice3/1, slice2/1, slice1/1
  slice16/1 -> reinterpret16/1
  reinterpret16/1 -> msb_out16/1
  slice15/1 -> reinterpret15/1
  reinterpret15/1 -> out15/1
  slice14/1 -> reinterpret14/1
  reinterpret14/1 -> out14/1
  slice13/1 -> reinterpret13/1
  reinterpret13/1 -> out13/1
  slice12/1 -> reinterpret12/1
  reinterpret12/1 -> out12/1
  slice11/1 -> reinterpret11/1
  reinterpret11/1 -> out11/1
  slice10/1 -> reinterpret10/1
  reinterpret10/1 -> out10/1
  slice9/1 -> reinterpret9/1
  reinterpret9/1 -> out9/1
  slice8/1 -> reinterpret8/1
  reinterpret8/1 -> out8/1
  slice7/1 -> reinterpret7/1
  reinterpret7/1 -> out7/1
  slice6/1 -> reinterpret6/1
  reinterpret6/1 -> out6/1
  slice5/1 -> reinterpret5/1
  reinterpret5/1 -> out5/1
  slice4/1 -> reinterpret4/1
  reinterpret4/1 -> out4/1
  slice3/1 -> reinterpret3/1
  reinterpret3/1 -> out3/1
  slice2/1 -> reinterpret2/1
  reinterpret2/1 -> out2/1
  slice1/1 -> reinterpret1/1
  reinterpret1/1 -> lsb_out1/1

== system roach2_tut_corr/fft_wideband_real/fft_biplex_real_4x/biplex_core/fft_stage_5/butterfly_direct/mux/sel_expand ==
  bus_in : Inport
  reinterpret{1..16} (16 alike) : xbsIndex_r4/Reinterpret  force_arith_type=on  arith_type=Unsigned  force_bin_pt=on  bin_pt=0  block_type=reinterpret
  slice1 : xbsIndex_r4/Slice  nbits=1  boolean_output=off  mode=Upper Bit Location + Width  bit1=-15  base1=MSB of Input  bit0=0  base0=LSB of Input  dbl_ovrd=off  block_type=slice
  slice10 : xbsIndex_r4/Slice  nbits=1  boolean_output=off  mode=Upper Bit Location + Width  bit1=-6  base1=MSB of Input  bit0=0  base0=LSB of Input  dbl_ovrd=off  block_type=slice
  slice11 : xbsIndex_r4/Slice  nbits=1  boolean_output=off  mode=Upper Bit Location + Width  bit1=-5  base1=MSB of Input  bit0=0  base0=LSB of Input  dbl_ovrd=off  block_type=slice
  slice12 : xbsIndex_r4/Slice  nbits=1  boolean_output=off  mode=Upper Bit Location + Width  bit1=-4  base1=MSB of Input  bit0=0  base0=LSB of Input  dbl_ovrd=off  block_type=slice
  slice13 : xbsIndex_r4/Slice  nbits=1  boolean_output=off  mode=Upper Bit Location + Width  bit1=-3  base1=MSB of Input  bit0=0  base0=LSB of Input  dbl_ovrd=off  block_type=slice
  slice14 : xbsIndex_r4/Slice  nbits=1  boolean_output=off  mode=Upper Bit Location + Width  bit1=-2  base1=MSB of Input  bit0=0  base0=LSB of Input  dbl_ovrd=off  block_type=slice
  slice15 : xbsIndex_r4/Slice  nbits=1  boolean_output=off  mode=Upper Bit Location + Width  bit1=-1  base1=MSB of Input  bit0=0  base0=LSB of Input  dbl_ovrd=off  block_type=slice
  slice16 : xbsIndex_r4/Slice  nbits=1  boolean_output=off  mode=Upper Bit Location + Width  bit1=0  base1=MSB of Input  bit0=0  base0=LSB of Input  dbl_ovrd=off  block_type=slice
  slice2 : xbsIndex_r4/Slice  nbits=1  boolean_output=off  mode=Upper Bit Location + Width  bit1=-14  base1=MSB of Input  bit0=0  base0=LSB of Input  dbl_ovrd=off  block_type=slice
  slice3 : xbsIndex_r4/Slice  nbits=1  boolean_output=off  mode=Upper Bit Location + Width  bit1=-13  base1=MSB of Input  bit0=0  base0=LSB of Input  dbl_ovrd=off  block_type=slice
  slice4 : xbsIndex_r4/Slice  nbits=1  boolean_output=off  mode=Upper Bit Location + Width  bit1=-12  base1=MSB of Input  bit0=0  base0=LSB of Input  dbl_ovrd=off  block_type=slice
  slice5 : xbsIndex_r4/Slice  nbits=1  boolean_output=off  mode=Upper Bit Location + Width  bit1=-11  base1=MSB of Input  bit0=0  base0=LSB of Input  dbl_ovrd=off  block_type=slice
  slice6 : xbsIndex_r4/Slice  nbits=1  boolean_output=off  mode=Upper Bit Location + Width  bit1=-10  base1=MSB of Input  bit0=0  base0=LSB of Input  dbl_ovrd=off  block_type=slice
  slice7 : xbsIndex_r4/Slice  nbits=1  boolean_output=off  mode=Upper Bit Location + Width  bit1=-9  base1=MSB of Input  bit0=0  base0=LSB of Input  dbl_ovrd=off  block_type=slice
  slice8 : xbsIndex_r4/Slice  nbits=1  boolean_output=off  mode=Upper Bit Location + Width  bit1=-8  base1=MSB of Input  bit0=0  base0=LSB of Input  dbl_ovrd=off  block_type=slice
  slice9 : xbsIndex_r4/Slice  nbits=1  boolean_output=off  mode=Upper Bit Location + Width  bit1=-7  base1=MSB of Input  bit0=0  base0=LSB of Input  dbl_ovrd=off  block_type=slice
  msb_out16 : Outport
  out15 : Outport  Port=2
  out14 : Outport  Port=3
  out13 : Outport  Port=4
  out12 : Outport  Port=5
  out11 : Outport  Port=6
  out10 : Outport  Port=7
  out9 : Outport  Port=8
  out8 : Outport  Port=9
  out7 : Outport  Port=10
  out6 : Outport  Port=11
  out5 : Outport  Port=12
  out4 : Outport  Port=13
  out3 : Outport  Port=14
  out2 : Outport  Port=15
  lsb_out1 : Outport  Port=16
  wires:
  bus_in/1 -> slice16/1, slice15/1, slice14/1, slice13/1, slice12/1, slice11/1, slice10/1, slice9/1, slice8/1, slice7/1, slice6/1, slice5/1, slice4/1, slice3/1, slice2/1, slice1/1
  slice16/1 -> reinterpret16/1
  reinterpret16/1 -> msb_out16/1
  slice15/1 -> reinterpret15/1
  reinterpret15/1 -> out15/1
  slice14/1 -> reinterpret14/1
  reinterpret14/1 -> out14/1
  slice13/1 -> reinterpret13/1
  reinterpret13/1 -> out13/1
  slice12/1 -> reinterpret12/1
  reinterpret12/1 -> out12/1
  slice11/1 -> reinterpret11/1
  reinterpret11/1 -> out11/1
  slice10/1 -> reinterpret10/1
  reinterpret10/1 -> out10/1
  slice9/1 -> reinterpret9/1
  reinterpret9/1 -> out9/1
  slice8/1 -> reinterpret8/1
  reinterpret8/1 -> out8/1
  slice7/1 -> reinterpret7/1
  reinterpret7/1 -> out7/1
  slice6/1 -> reinterpret6/1
  reinterpret6/1 -> out6/1
  slice5/1 -> reinterpret5/1
  reinterpret5/1 -> out5/1
  slice4/1 -> reinterpret4/1
  reinterpret4/1 -> out4/1
  slice3/1 -> reinterpret3/1
  reinterpret3/1 -> out3/1
  slice2/1 -> reinterpret2/1
  reinterpret2/1 -> out2/1
  slice1/1 -> reinterpret1/1
  reinterpret1/1 -> lsb_out1/1

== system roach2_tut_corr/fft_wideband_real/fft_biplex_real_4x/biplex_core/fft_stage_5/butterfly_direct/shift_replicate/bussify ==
  in1 : Inport
  in2 : Inport  Port=2
  in3 : Inport  Port=3
  in4 : Inport  Port=4
  in5 : Inport  Port=5
  in6 : Inport  Port=6
  in7 : Inport  Port=7
  in8 : Inport  Port=8
  in9 : Inport  Port=9
  in10 : Inport  Port=10
  in11 : Inport  Port=11
  in12 : Inport  Port=12
  in13 : Inport  Port=13
  in14 : Inport  Port=14
  in15 : Inport  Port=15
  in16 : Inport  Port=16
  concatenate : xbsIndex_r4/Concat  num_inputs=16  dbl_ovrd=off  block_type=concat
  reinterpret{1..16} (16 alike) : xbsIndex_r4/Reinterpret  force_arith_type=on  arith_type=Unsigned  force_bin_pt=on  bin_pt=0  block_type=reinterpret
  bus_out : Outport
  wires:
  concatenate/1 -> bus_out/1
  in1/1 -> reinterpret1/1
  reinterpret1/1 -> concatenate/1
  in2/1 -> reinterpret2/1
  reinterpret2/1 -> concatenate/2
  in3/1 -> reinterpret3/1
  reinterpret3/1 -> concatenate/3
  in4/1 -> reinterpret4/1
  reinterpret4/1 -> concatenate/4
  in5/1 -> reinterpret5/1
  reinterpret5/1 -> concatenate/5
  in6/1 -> reinterpret6/1
  reinterpret6/1 -> concatenate/6
  in7/1 -> reinterpret7/1
  reinterpret7/1 -> concatenate/7
  in8/1 -> reinterpret8/1
  reinterpret8/1 -> concatenate/8
  in9/1 -> reinterpret9/1
  reinterpret9/1 -> concatenate/9
  in10/1 -> reinterpret10/1
  reinterpret10/1 -> concatenate/10
  in11/1 -> reinterpret11/1
  reinterpret11/1 -> concatenate/11
  in12/1 -> reinterpret12/1
  reinterpret12/1 -> concatenate/12
  in13/1 -> reinterpret13/1
  reinterpret13/1 -> concatenate/13
  in14/1 -> reinterpret14/1
  reinterpret14/1 -> concatenate/14
  in15/1 -> reinterpret15/1
  reinterpret15/1 -> concatenate/15
  in16/1 -> reinterpret16/1
  reinterpret16/1 -> concatenate/16

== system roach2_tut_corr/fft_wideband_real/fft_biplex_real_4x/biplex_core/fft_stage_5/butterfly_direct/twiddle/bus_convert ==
  din : Inport
  misci : Inport  Port=2
  bussify : Subsystem  AncestorBlock=casper_library_flow_control/bus_create
  conv1 : Subsystem  AncestorBlock=casper_library_misc/convert
  conv2 : Subsystem  AncestorBlock=casper_library_misc/convert
  conv3 : Subsystem  AncestorBlock=casper_library_misc/convert
  conv4 : Subsystem  AncestorBlock=casper_library_misc/convert
  conv5 : Subsystem  AncestorBlock=casper_library_misc/convert
  conv6 : Subsystem  AncestorBlock=casper_library_misc/convert
  conv7 : Subsystem  AncestorBlock=casper_library_misc/convert
  conv8 : Subsystem  AncestorBlock=casper_library_misc/convert
  debus : Subsystem  AncestorBlock=casper_library_flow_control/bus_expand
  dmisc : xbsIndex_r4/Delay  rst=off  infoeditControl=Selection of Reset will increase slice count due to use of real FFs and instead of SRLs  en=off  latency=latency  dbl_ovrd=off  reg_retiming=on  block_type=delay
  dout : Outport
  misco : Outport  Port=2
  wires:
  din/1 -> debus/1(bus_in)
  debus/1(msb_out8) -> conv1/1(in)
  debus/2(out7) -> conv2/1(in)
  debus/3(out6) -> conv3/1(in)
  debus/4(out5) -> conv4/1(in)
  debus/5(out4) -> conv5/1(in)
  debus/6(out3) -> conv6/1(in)
  debus/7(out2) -> conv7/1(in)
  debus/8(lsb_out1) -> conv8/1(in)
  misci/1 -> dmisc/1
  conv1/1(out) -> bussify/1(in1)
  conv2/1(out) -> bussify/2(in2)
  conv3/1(out) -> bussify/3(in3)
  conv4/1(out) -> bussify/4(in4)
  conv5/1(out) -> bussify/5(in5)
  conv6/1(out) -> bussify/6(in6)
  conv7/1(out) -> bussify/7(in7)
  conv8/1(out) -> bussify/8(in8)
  bussify/1(bus_out) -> dout/1
  dmisc/1 -> misco/1

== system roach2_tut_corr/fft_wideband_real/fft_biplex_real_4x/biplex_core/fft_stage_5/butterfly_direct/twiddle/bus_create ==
  in1 : Inport
  in2 : Inport  Port=2
  in3 : Inport  Port=3
  concatenate : xbsIndex_r4/Concat  num_inputs=3  dbl_ovrd=off  block_type=concat
  reinterpret1 : xbsIndex_r4/Reinterpret  force_arith_type=on  arith_type=Unsigned  force_bin_pt=on  bin_pt=0  block_type=reinterpret
  reinterpret2 : xbsIndex_r4/Reinterpret  force_arith_type=on  arith_type=Unsigned  force_bin_pt=on  bin_pt=0  block_type=reinterpret
  reinterpret3 : xbsIndex_r4/Reinterpret  force_arith_type=on  arith_type=Unsigned  force_bin_pt=on  bin_pt=0  block_type=reinterpret
  bus_out : Outport
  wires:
  concatenate/1 -> bus_out/1
  in1/1 -> reinterpret1/1
  reinterpret1/1 -> concatenate/1
  in2/1 -> reinterpret2/1
  reinterpret2/1 -> concatenate/2
  in3/1 -> reinterpret3/1
  reinterpret3/1 -> concatenate/3

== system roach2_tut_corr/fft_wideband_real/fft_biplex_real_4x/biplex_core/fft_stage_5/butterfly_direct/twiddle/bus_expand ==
  bus_in : Inport
  reinterpret1 : xbsIndex_r4/Reinterpret  force_arith_type=on  arith_type=Unsigned  force_bin_pt=on  bin_pt=0  block_type=reinterpret
  reinterpret2 : xbsIndex_r4/Reinterpret  force_arith_type=on  arith_type=Unsigned  force_bin_pt=on  bin_pt=0  block_type=reinterpret
  slice1 : xbsIndex_r4/Slice  nbits=145  boolean_output=off  mode=Upper Bit Location + Width  bit1=-144  base1=MSB of Input  bit0=0  base0=LSB of Input  dbl_ovrd=off  block_type=slice
  slice2 : xbsIndex_r4/Slice  nbits=144  boolean_output=off  mode=Upper Bit Location + Width  bit1=0  base1=MSB of Input  bit0=0  base0=LSB of Input  dbl_ovrd=off  block_type=slice
  msb_out2 : Outport
  lsb_out1 : Outport  Port=2
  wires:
  bus_in/1 -> slice2/1, slice1/1
  slice2/1 -> reinterpret2/1
  reinterpret2/1 -> msb_out2/1
  slice1/1 -> reinterpret1/1
  reinterpret1/1 -> lsb_out1/1

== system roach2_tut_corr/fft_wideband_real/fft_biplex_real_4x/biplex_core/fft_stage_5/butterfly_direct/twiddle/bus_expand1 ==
  bus_in : Inport
  reinterpret1 : xbsIndex_r4/Reinterpret  force_arith_type=on  arith_type=Unsigned  force_bin_pt=on  bin_pt=0  block_type=reinterpret
  slice1 : xbsIndex_r4/Slice  nbits=144  boolean_output=off  mode=Upper Bit Location + Width  bit1=-1  base1=MSB of Input  bit0=0  base0=LSB of Input  dbl_ovrd=off  block_type=slice
  slice2 : xbsIndex_r4/Slice  nbits=1  boolean_output=on  mode=Upper Bit Location + Width  bit1=0  base1=MSB of Input  bit0=0  base0=LSB of Input  dbl_ovrd=off  block_type=slice
  msb_out2 : Outport
  lsb_out1 : Outport  Port=2
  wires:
  bus_in/1 -> slice2/1, slice1/1
  slice2/1 -> msb_out2/1
  slice1/1 -> reinterpret1/1
  reinterpret1/1 -> lsb_out1/1

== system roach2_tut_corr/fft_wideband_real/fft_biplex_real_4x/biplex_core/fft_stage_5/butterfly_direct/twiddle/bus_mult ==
  a : Inport
  b : Inport  Port=2
  misci : Inport  Port=3
  a*b_bussify : Subsystem  AncestorBlock=casper_library_flow_control/bus_create
  a_debus : Subsystem  AncestorBlock=casper_library_flow_control/bus_expand
  b_debus : Subsystem  AncestorBlock=casper_library_flow_control/bus_expand
  dmisc : xbsIndex_r4/Delay  rst=off  infoeditControl=Selection of Reset will increase slice count due to use of real FFs and instead of SRLs  en=off  latency=mult_latency+add_latency+conv_latency+fan_latency  dbl_ovrd=off  reg_retiming=on  block_type=delay
  mult1 : Subsystem  AncestorBlock=casper_library_multipliers/cmult
  mult2 : Subsystem  AncestorBlock=casper_library_multipliers/cmult
  mult3 : Subsystem  AncestorBlock=casper_library_multipliers/cmult
  mult4 : Subsystem  AncestorBlock=casper_library_multipliers/cmult
  repa : Subsystem  AncestorBlock=casper_library_bus/bus_replicate
  repb : Subsystem  AncestorBlock=casper_library_bus/bus_replicate
  a*b : Outport
  misco : Outport  Port=2
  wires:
  a/1 -> repa/1(in)
  b/1 -> repb/1(in)
  repa/1(out) -> a_debus/1(bus_in)
  repb/1(out) -> b_debus/1(bus_in)
  a_debus/1(msb_lsb_out1) -> mult1/1(a), mult2/1(a), mult3/1(a), mult4/1(a)
  b_debus/1(msb_out4) -> mult1/2(b)
  b_debus/2(out3) -> mult2/2(b)
  b_debus/3(out2) -> mult3/2(b)
  b_debus/4(lsb_out1) -> mult4/2(b)
  misci/1 -> dmisc/1
  mult1/1(ab) -> a*b_bussify/1(in1)
  mult2/1(ab) -> a*b_bussify/2(in2)
  mult3/1(ab) -> a*b_bussify/3(in3)
  mult4/1(ab) -> a*b_bussify/4(in4)
  a*b_bussify/1(bus_out) -> a*b/1
  dmisc/1 -> misco/1

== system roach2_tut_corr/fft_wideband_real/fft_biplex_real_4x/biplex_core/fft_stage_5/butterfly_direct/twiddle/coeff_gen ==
  rst : Inport
  misci : Inport  Port=2
  Counter : xbsIndex_r4/Counter  cnt_type=Free Running  cnt_to=Inf  operation=Up  start_count=0  cnt_by_val=1  arith_type=Unsigned  n_bits=8  bin_pt=0  load_pin=off  rst=on  en=off  explicit_period=on  period=1  dbl_ovrd=off  use_behavioral_HDL=on  implementation=Fabric  block_type=counter
  Slice : xbsIndex_r4/Slice  nbits=4  boolean_output=off  mode=Upper Bit Location + Width  bit1=0  base1=MSB of Input  bit0=0  base0=LSB of Input  dbl_ovrd=off  block_type=slice
  bit_reverse : Subsystem  AncestorBlock=casper_library_misc/bit_reverse
  cosin : Subsystem  Tag=casper:cosin  AncestorBlock=casper_library_downconverter/cosin
  ri_to_c : casper_library_misc/ri_to_c
  w : Outport
  misco : Outport  Port=2
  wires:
  ri_to_c/1 -> w/1
  rst/1 -> Counter/1
  Counter/1 -> Slice/1
  Slice/1 -> bit_reverse/1(in)
  bit_reverse/1(out) -> cosin/1(theta)
  cosin/1(cos) -> ri_to_c/1
  cosin/2(-sin) -> ri_to_c/2
  misci/1 -> cosin/2(misci)
  cosin/3(misco) -> misco/1
